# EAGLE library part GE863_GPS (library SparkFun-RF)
GE863 Cellular Module with GPS Proto layout and schematic for GE863 cellular module with SiRF III GPS. Spark Fun Electronics SKU : CEL-08246
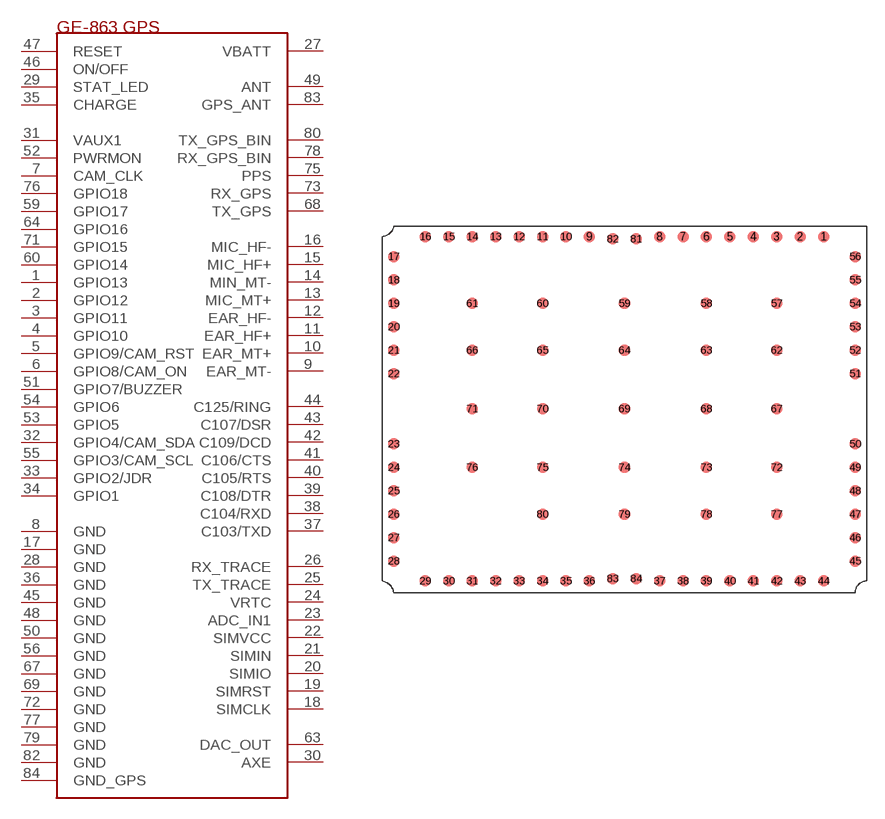
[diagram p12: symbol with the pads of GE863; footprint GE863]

Designator prefix -

## GE863_GPS  [GE863]
1  GPIO13
2  GPIO12
3  GPIO11
4  GPIO10
5  GPIO9/CAM_RST
6  GPIO8/CAM_ON
7  CAM_CLK
8  GND
9  EAR_MT-
10  EAR_MT+
11  EAR_HF+
12  EAR_HF-
13  MIC_MT+
14  MIN_MT-
15  MIC_HF+
16  MIC_HF-
17  GND
18  SIMCLK
19  SIMRST
20  SIMIO
21  SIMIN
22  SIMVCC
23  ADC_IN1
24  VRTC
25  TX_TRACE
26  RX_TRACE
27  VBATT
28  GND
29  STAT_LED
30  AXE
31  VAUX1
32  GPIO4/CAM_SDA
33  GPIO2/JDR
34  GPIO1
35  CHARGE
36  GND
37  C103/TXD
38  C104/RXD
39  C108/DTR
40  C105/RTS
41  C106/CTS
42  C109/DCD
43  C107/DSR
44  C125/RING
45  GND
46  ON/OFF
47  RESET
48  GND
49  ANT
50  GND
51  GPIO7/BUZZER
52  PWRMON
53  GPIO5
54  GPIO6
55  GPIO3/CAM_SCL
56  GND
59  GPIO17
60  GPIO14
63  DAC_OUT
64  GPIO16
67  GND
68  TX_GPS
69  GND
71  GPIO15
72  GND
73  RX_GPS
75  PPS
76  GPIO18
77  GND
78  RX_GPS_BIN
79  GND
80  TX_GPS_BIN
82  GND
83  GPS_ANT
84  GND_GPS

## Footprint GE863 (pad centres in mm)
smd 1 x 1: 1 17,14.7; 2 15,14.7; 3 13,14.7; 4 11,14.7; 5 9,14.7; 6 7,14.7; 7 5,14.7; 8 3,14.7; 9 -3,14.7; 10 -5,14.7; 11 -7,14.7; 12 -9,14.7; 13 -11,14.7; 14 -13,14.7; 15 -15,14.7; 16 -17,14.7; 17 -19.7,13; 18 -19.7,11; 19 -19.7,9; 20 -19.7,7; 21 -19.7,5; 22 -19.7,3; 23 -19.7,-3; 24 -19.7,-5; 25 -19.7,-7; 26 -19.7,-9; 27 -19.7,-11; 28 -19.7,-13; 29 -17,-14.7; 30 -15,-14.7; 31 -13,-14.7; 32 -11,-14.7; 33 -9,-14.7; 34 -7,-14.7; 35 -5,-14.7; 36 -3,-14.7; 37 3,-14.7; 38 5,-14.7; 39 7,-14.7; 40 9,-14.7; 41 11,-14.7; 42 13,-14.7; 43 15,-14.7; 44 17,-14.7; 45 19.7,-13; 46 19.7,-11; 47 19.7,-9; 48 19.7,-7; 49 19.7,-5; 50 19.7,-3; 51 19.7,3; 52 19.7,5; 53 19.7,7; 54 19.7,9; 55 19.7,11; 56 19.7,13; 57 13,9; 58 7,9; 59 0,9; 60 -7,9; 61 -13,9; 62 13,5; 63 7,5; 64 0,5; 65 -7,5; 66 -13,5; 67 13,0; 68 7,0; 69 0,0; 70 -7,0; 71 -13,0; 72 13,-5; 73 7,-5; 74 0,-5; 75 -7,-5; 76 -13,-5; 77 13,-9; 78 7,-9; 79 0,-9; 80 -7,-9; 81 1,14.5; 82 -1,14.5; 83 -1,-14.5; 84 1,-14.5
